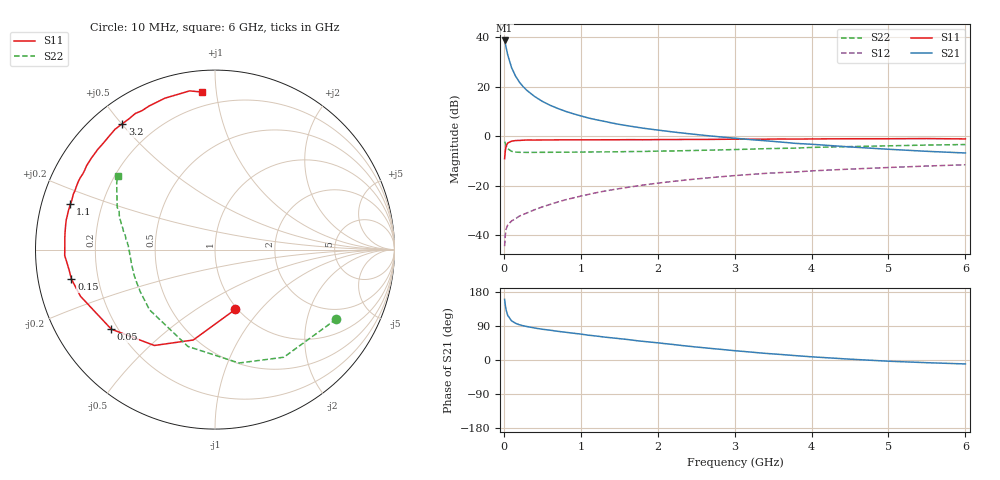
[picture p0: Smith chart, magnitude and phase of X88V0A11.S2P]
! SIEMENS Small Signal Semiconductors
! BFP136W
! Si NPN RF Bipolar Junction Transistor in SOT343
! VCE = 8 V  IC = 110 mA
! Common Emitter S-Parameters:  September  1994
# GHz  S  MA  R  50
!  f  S11  S21  S12  S22
! GHz  MAG  ANG  MAG  ANG  MAG  ANG  MAG  ANG
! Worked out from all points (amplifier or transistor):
!   40 points, 10 MHz to 6 GHz, reference 50 ohm
!   highest |S21| = 38.7 dB at 10 MHz (marker M1)
!   |S21| within 3 dB of that: start of sweep to 31.1 MHz
!   unconditionally stable (mu >= 1): 591 MHz to 2.977 GHz; 3.105 GHz to 3.258 GHz
!   at 200 MHz: K = 0.66, MSG = 27.1 dB, |S12| = -32.3 dB
!   at 1.5 GHz: K = 1.11, MAG = 11.0 dB, |S12| = -21.2 dB
!   at 6 GHz: K = 0.97, MSG = 2.4 dB, |S12| = -11.5 dB
!   S11 on the Smith chart (normalised r, x): 10 MHz: 0.98, -0.74; 50 MHz: 0.17, -0.33; 150 MHz: 0.10, -0.10; 1.1 GHz: 0.09, +0.15; 3.2 GHz: 0.09, +0.50; 6 GHz: 0.12, +0.91
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0.01  0.3517 -71.2  86.05 160.0  0.006 68.4  0.779 -29.8
0.02  0.5179 -103.5  73.51 143.6  0.0103 56.4  0.7118 -57.4
0.03  0.632 -122.3  62.06 131.9  0.0133 49.7  0.6459 -78.0
0.05  0.7283 -142.5  44.22 117.9  0.016 38.1  0.5603 -105.6
0.1  0.7934 -160.9  24.43 103.4  0.0194 35.7  0.4957 -137.4
0.15  0.8165 -168.3  16.62 97.1  0.0215 38.0  0.478 -150.6
0.2  0.8213 -172.3  12.5 93.2  0.0242 39.6  0.473 -157.8
0.25  0.8302 -175.6  10.07 90.4  0.0262 42.4  0.4726 -162.4
0.3  0.838 -177.7  8.432 88.3  0.0281 44.4  0.471 -165.5
0.4  0.8371 178.3  6.349 84.4  0.0327 48.7  0.4719 -169.6
0.5  0.8392 175.5  5.063 81.2  0.0373 51.1  0.4722 -172.5
0.6  0.841 173.3  4.229 78.7  0.0418 53.6  0.4731 -174.4
0.7  0.8432 170.7  3.645 75.7  0.0468 55.6  0.4745 -175.7
0.9  0.8444 167.0  2.85 70.8  0.0565 57.0  0.4765 -178.3
1.1  0.8443 162.6  2.333 65.4  0.0667 58.1  0.4796 -180.0
1.5  0.8483 155.8  1.734 56.4  0.0872 57.8  0.4852 176.9
1.8  0.8487 150.1  1.462 49.4  0.1025 56.2  0.4916 174.7
2.2  0.8568 143.5  1.218 40.9  0.1223 53.5  0.5033 171.8
3.2  0.8708 126.4  0.855 21.1  0.1685 44.9  0.5472 163.4
4.5  0.8886 108.3  0.607 2.2  0.2165 33.7  0.6166 152.3
5.5  0.8956 99.1  0.495 -7.1  0.2494 25.5  0.6622 145.8
6  0.8811 94.8  0.458 -10.4  0.2653 21.3  0.6791 142.9
